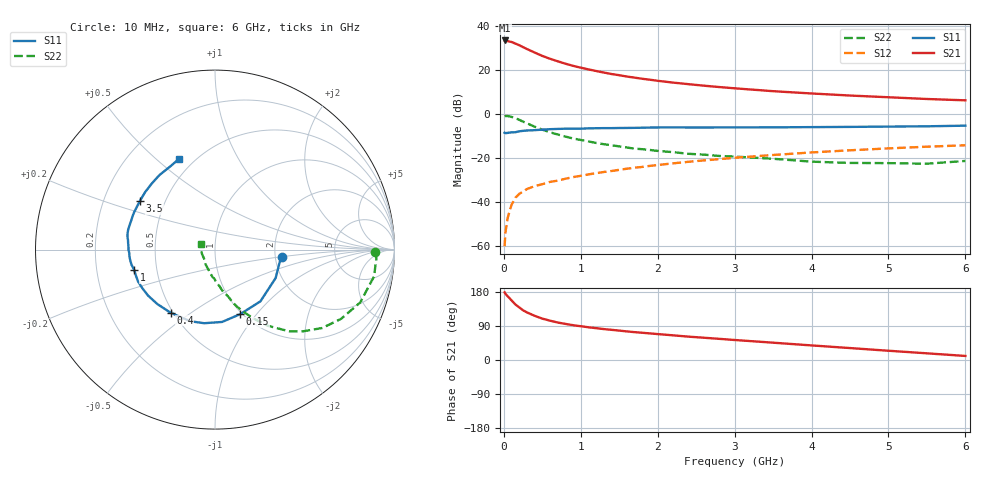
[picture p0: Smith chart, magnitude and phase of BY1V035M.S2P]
! SIEMENS Small Signal Semiconductors
! BFY420
! Si NPN RF SIEGET Grounded Emitter Transistor in MICRO-X
! VCE = 1 V  IC = 35 mA
! Common Emitter S-Parameters:  October  1996
# GHz  S  MA  R  50
!  f  S11  S21  S12  S22
! GHz  MAG  ANG  MAG  ANG  MAG  ANG  MAG  ANG
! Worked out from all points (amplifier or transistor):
!   36 points, 10 MHz to 6 GHz, reference 50 ohm
!   highest |S21| = 33.4 dB at 10 MHz (marker M1)
!   |S21| within 3 dB of that: start of sweep to 248.3 MHz
!   unconditionally stable (mu >= 1): start of sweep to 18.34 MHz; 1.257 GHz to end of sweep
!   at 250 MHz: K = 0.43, MSG = 32.8 dB, |S12| = -35.2 dB
!   at 1.4 GHz: K = 1.04, MAG = 20.8 dB, |S12| = -25.9 dB
!   at 6 GHz: K = 1.10, MAG = 8.3 dB, |S12| = -14.2 dB
!   S11 on the Smith chart (normalised r, x): 10 MHz: 2.18, -0.21; 150 MHz: 0.98, -0.83; 400 MHz: 0.48, -0.42; 1 GHz: 0.37, -0.11; 3.5 GHz: 0.36, +0.26; 6 GHz: 0.42, +0.60
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0.01  0.376 -6.3  46.74 178.3  0.001 115.7  0.8906 -0.9
0.02  0.3672 -10.7  46.53 174.7  0.002 81.8  0.9007 -3.0
0.05  0.3731 -25.1  45.13 168.1  0.0044 86.9  0.8985 -9.6
0.1  0.3836 -48.7  43.13 157.4  0.0087 76.5  0.861 -20.0
0.15  0.3861 -68.7  39.78 146.6  0.0126 68.0  0.8013 -28.8
0.2  0.405 -84.4  36.51 138.8  0.0154 66.2  0.7397 -36.2
0.25  0.4146 -98.4  32.97 131.2  0.0173 62.6  0.6708 -42.7
0.3  0.4222 -109.1  29.91 125.5  0.0198 60.7  0.6161 -47.7
0.4  0.43 -125.2  24.87 116.7  0.023 58.3  0.5158 -55.3
0.5  0.4419 -136.7  20.82 109.2  0.0255 57.6  0.4411 -60.7
0.6  0.4525 -145.5  17.97 103.8  0.0288 57.0  0.3856 -65.0
0.7  0.4585 -152.1  15.73 98.9  0.0307 57.3  0.3426 -68.7
0.8  0.464 -157.5  13.88 95.3  0.0339 57.5  0.3074 -71.7
1  0.4644 -166.0  11.26 89.1  0.0395 58.3  0.2576 -76.1
1.1  0.4728 -169.7  10.31 86.3  0.0426 58.9  0.2386 -79.1
1.4  0.4781 -177.8  8.08 79.6  0.0508 59.5  0.1955 -85.0
1.6  0.4825 178.0  7.087 75.4  0.0573 58.7  0.1733 -89.3
2.2  0.4963 167.1  5.165 65.1  0.0759 56.1  0.1363 -100.5
3.5  0.4985 147.2  3.298 45.7  0.1174 47.1  0.0964 -123.8
4.5  0.5098 133.4  2.626 31.5  0.1501 37.7  0.0776 -144.3
5.5  0.5263 118.2  2.193 17.6  0.1811 27.3  0.0745 176.4
6  0.5436 111.7  2.044 10.7  0.1951 22.1  0.086 157.7
